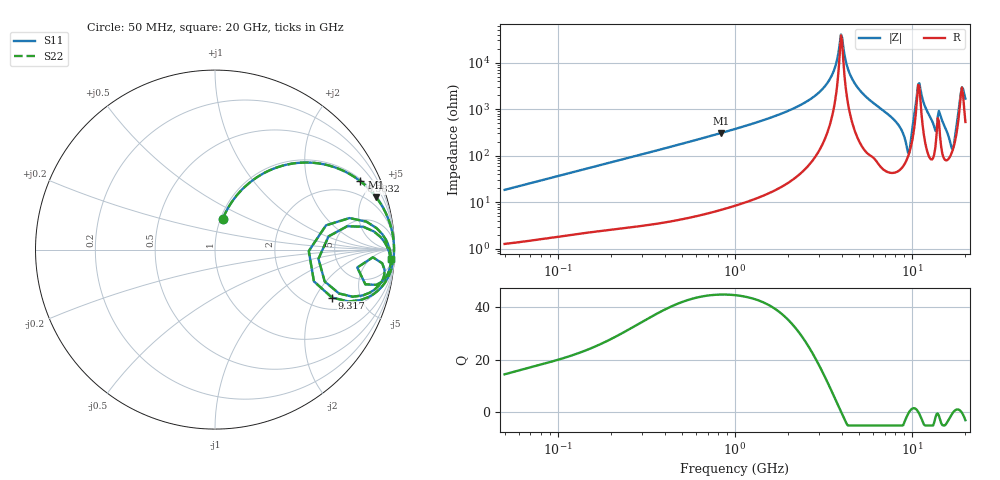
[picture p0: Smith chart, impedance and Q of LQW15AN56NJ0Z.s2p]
!Murata Part Number: LQW15AN56NJ0Z
!These Parameters are Measured in Series Mode Connection
!  o--[Z]--o
!Port1  Port2
!  o-------o
!Freq. Start=50[MHz] Stop=20[GHz], 401[Steps]
# Hz S RI R 50
!Freq.(Hz) S11(Real) S11(Imag) S21(Real) S21(Imag) S12(Real) S12(Imag) S22(Real) S22(Imag)
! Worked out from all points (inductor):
!   401 points, 50 MHz to 20 GHz, reference 50 ohm
!   read as one part in series: L = 58.2 nH near 51.52 MHz
!   highest Q = 44.8 at 835.5 MHz (marker M1), where L = 58.4 nH
!   self-resonance near 3.967 GHz
!   S11 on the Smith chart (normalised r, x): 50 MHz: 1.03, +0.37; 583.2 MHz: 1.10, +4.20; 9.317 GHz: 2.61, -2.77; 20 GHz: 12, -32
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5e7  0.0439 0.1733  0.9561 -0.1733  0.9561 -0.1733  0.0439 0.1733
1.364002e8  0.2048 0.3824  0.7952 -0.3824  0.7952 -0.3824  0.2048 0.3824
3.721004e8  0.6353 0.4684  0.3647 -0.4684  0.3647 -0.4684  0.6353 0.4684
5.831961e8  0.8098 0.3811  0.1902 -0.3811  0.1902 -0.3811  0.8098 0.3811
8.354841e8  0.8987 0.2908  0.1013 -0.2908  0.1013 -0.2908  0.8987 0.2908
1e9  0.9284 0.2469  0.0716 -0.2469  0.0716 -0.2469  0.9284 0.2469
2.728004e9  0.9942 0.0569  0.00578 -0.0569  0.00578 -0.0569  0.9942 0.0569
3.466789e9  0.9972 0.021  0.0028 -0.021  0.0028 -0.021  0.9972 0.021
3.967106e9  0.9976 0.000665  0.00239 -0.000665  0.00239 -0.000665  0.9976 0.000665
4.81993e9  0.9963 -0.0303  0.00366 0.0303  0.00366 0.0303  0.9963 -0.0303
7.442007e9  0.9742 -0.1317  0.0258 0.1317  0.0258 0.1317  0.9742 -0.1317
8.644534e9  0.907 -0.2295  0.093 0.2295  0.093 0.2295  0.907 -0.2295
9.316812e9  0.6518 -0.2673  0.3482 0.2673  0.3482 0.2673  0.6518 -0.2673
1.004137e10  0.8433 0.1557  0.1567 -0.1557  0.1567 -0.1557  0.8433 0.1557
1.066139e10  0.9648 0.028  0.0352 -0.028  0.0352 -0.028  0.9648 0.028
1.098561e10  0.9762 -0.013  0.0238 0.013  0.0238 0.013  0.9762 -0.013
1.314879e10  0.9298 -0.1795  0.0702 0.1795  0.0702 0.1795  0.9298 -0.1795
1.438523e10  0.9445 -0.1108  0.0555 0.1108  0.0555 0.1108  0.9445 -0.1108
1.670968e10  0.611 -0.1774  0.389 0.1774  0.389 0.1774  0.611 -0.1774
1.747767e10  0.7363 0.13  0.2637 -0.13  0.2637 -0.13  0.7363 0.13
1.88369e10  0.9588 0.0164  0.0412 -0.0164  0.0412 -0.0164  0.9588 0.0164
2e10  0.9785 -0.0544  0.0215 0.0544  0.0215 0.0544  0.9785 -0.0544
